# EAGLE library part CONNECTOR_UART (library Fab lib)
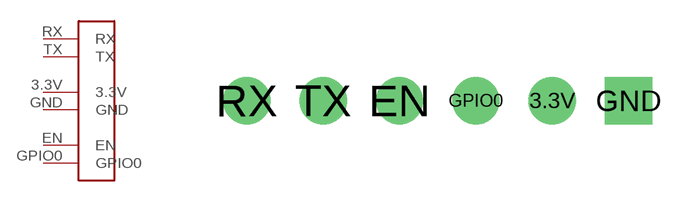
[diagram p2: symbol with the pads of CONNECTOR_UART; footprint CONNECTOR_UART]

Designator prefix -

## CONNECTOR_UART  [CONNECTOR_UART]
3.3V  3.3V
EN  EN
GND  GND
GPIO0  GPIO0
RX  RX
TX  TX

## Footprint CONNECTOR_UART (pad centres in mm)
drill 1.05: 3.3V 10.16,0; EN 5.08,0; GPIO0 7.62,0; RX 0,0; TX 2.54,0
drill 1.05 square: GND 12.7,0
